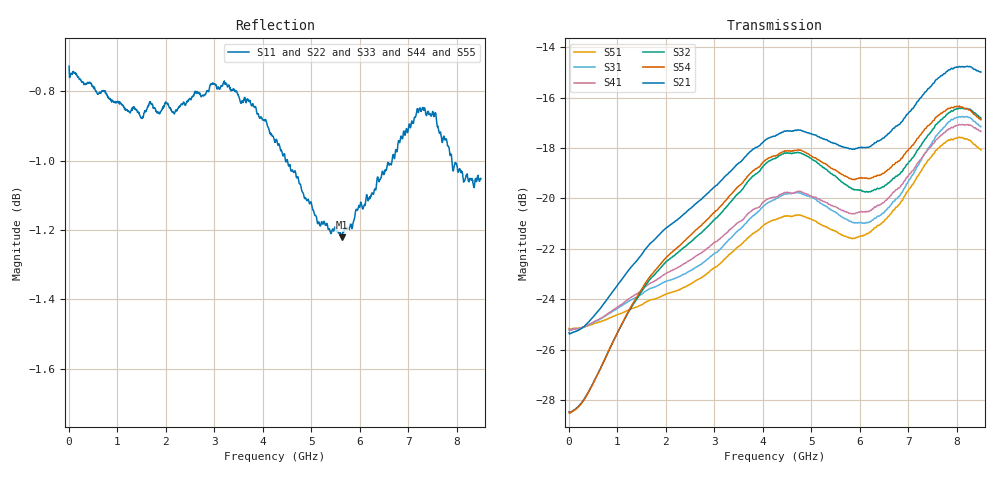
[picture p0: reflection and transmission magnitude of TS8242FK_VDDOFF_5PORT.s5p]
! Created with skrf (http://scikit-rf.org).
# Hz S RI R 50.0
!freq ReS11 ImS11 ReS12 ImS12 ReS13 ImS13
! ReS14 ImS14 ReS15 ImS15
! ReS21 ImS21 ReS22 ImS22 ReS23 ImS23
! ReS24 ImS24 ReS25 ImS25
! ReS31 ImS31 ReS32 ImS32 ReS33 ImS33
! ReS34 ImS34 ReS35 ImS35
! ReS41 ImS41 ReS42 ImS42 ReS43 ImS43
! ReS44 ImS44 ReS45 ImS45
! ReS51 ImS51 ReS52 ImS52 ReS53 ImS53
! ReS54 ImS54 ReS55 ImS55
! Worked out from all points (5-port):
!   1601 points, 10 MHz to 8.5 GHz, reference 50 ohm
!   strongest paths, dB at 10 MHz, 2.132 GHz, 4.255 GHz, 6.378 GHz, 8.5 GHz:
!     S21: -25.3, -21.0, -17.5, -17.7, -15.0
!     S54: -28.5, -22.1, -18.3, -19.1, -16.9
!     S32: -28.5, -22.3, -18.4, -19.6, -16.8
!     S41: -25.2, -22.9, -20.0, -20.3, -17.3
!     S31: -25.2, -23.2, -20.0, -20.7, -17.2
!     S51: -25.1, -23.7, -20.9, -21.1, -18.1
!   lowest |S11| = -1.2 dB at 5.629 GHz (marker M1), VSWR 14.25, Z = 6.82 + j48.4 ohm
!   |S11| at or under -10 dB: nowhere
